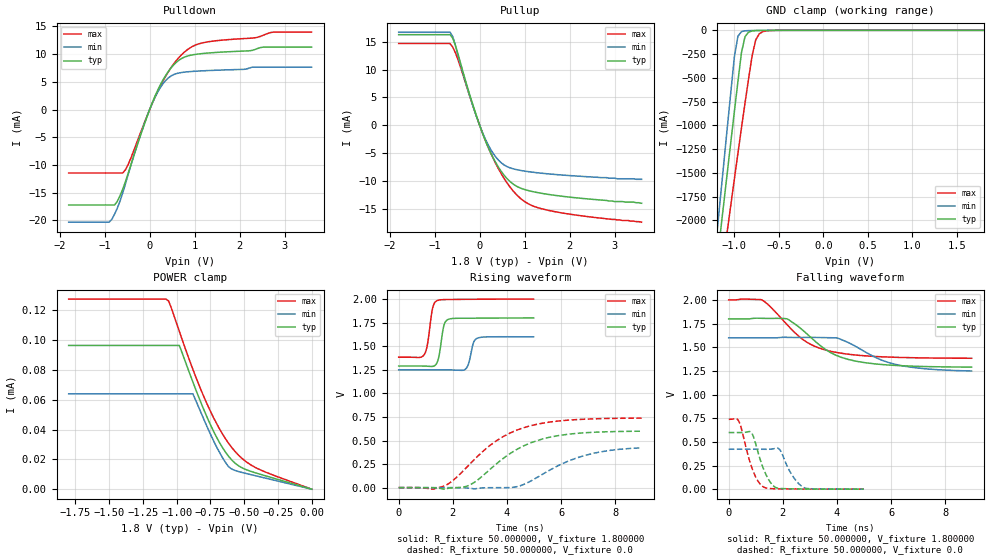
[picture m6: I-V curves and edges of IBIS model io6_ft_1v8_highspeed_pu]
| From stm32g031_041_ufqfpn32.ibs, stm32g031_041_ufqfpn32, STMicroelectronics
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|   Model io6_ft_1v8_highspeed_pu
[Model]  io6_ft_1v8_highspeed_pu
Model_type I/O
Polarity   Non-Inverting
Enable   Active-Low
Vinl =   0.540000V
Vinh =   1.260000V
Vmeas =  0.900000V
Cref =   50.000000pF
Rref =   100.000000M
Vref =   0.0V
C_comp   1.277600pF   1.236700pF   1.315100pF
[Temperature Range]   25.000000   -40.000000   0.125000k
[Pullup Reference]   1.800000V   1.600000V   2.000000V
[Pulldown Reference]   0.0V   0.0V   0.0V
[POWER Clamp Reference]   1.800000V   1.600000V   2.000000V
[GND Clamp Reference]   0.0V   0.0V   0.0V
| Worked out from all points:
|   slope of the pulldown table from 0 to 0.27 V, typ, clamps not added: 54.7 ohm
|   slope of the pullup table from 0 to 0.27 V, typ, clamps not added: 50.6 ohm
|   GND clamp passes 1 mA (typ) near -0.66 V on its own axis
|   rising waveform, R_fixture 50.000000, V_fixture 1.800000: 20-80 % time 166ps typ, 169ps min, 180ps max; typ from 1.29 V to 1.8 V
|   rising waveform, R_fixture 50.000000, V_fixture 0.0: 20-80 % time 1.83ns typ, 1.86ns min, 1.92ns max; typ from 0.001 V to 0.599 V
|   falling waveform, R_fixture 50.000000, V_fixture 1.800000: 20-80 % time 1.51ns typ, 1.6ns min, 1.49ns max; typ from 1.8 V to 1.29 V
|   falling waveform, R_fixture 50.000000, V_fixture 0.0: 20-80 % time 441ps typ, 482ps min, 451ps max; typ from 0.599 V to 0.001 V
[Pulldown]
|Voltage   I(typ)   I(min)   I(max)
-1.8V     -17.22mA   -20.33mA   -11.45mA
-900mV    -17.22mA   -20.33mA   -11.45mA
-720mV    -16.58mA   -17.82mA   -11.45mA
-600mV    -14.41mA   -15.08mA   -11.45mA
-480mV    -11.58mA   -11.79mA   -9.955mA
0V        0A         0A         0A
240mV     4.49mA     3.999mA    4.291mA
480mV     7.563mA    6.085mA    7.612mA
780mV     9.487mA    6.76mA     10.43mA
1.14V     10.08mA    6.976mA    11.96mA
2.76V     11.26mA    7.647mA    13.98mA
3.6V      11.26mA    7.647mA    13.98mA
[Pullup]
|Voltage   I(typ)   I(min)   I(max)
-1.8V     16.27mA    16.74mA    14.68mA
-660mV    16.27mA    16.74mA    14.68mA
-600mV    15.66mA    15.96mA    14.07mA
-480mV    12.75mA    12.58mA    11.77mA
-180mV    4.421mA    4.232mA    4.226mA
120mV     -2.604mA   -2.366mA   -2.563mA
420mV     -7.546mA   -6.272mA   -7.834mA
600mV     -9.499mA   -7.385mA   -10.25mA
780mV     -10.75mA   -7.883mA   -12.12mA
1.08V     -11.72mA   -8.32mA    -14.1mA
1.5V      -12.38mA   -8.703mA   -15.22mA
3.6V      -14mA      -9.7mA     -17.4mA
[GND_clamp]
|Voltage   I(typ)   I(min)   I(max)
-1.8V     -7.471A    -7.973A    -7.298A
-1.2V     -2.489A    -2.18A     -2.954A
-1.16V    -2.16A     -1.797A    -2.674A
-1.08V    -1.505A    -1.034A    -2.118A
-1V       -857.9mA   -283.1mA   -1.568A
-960mV    -540.4mA   -62.14mA   -1.296A
-920mV    -234.4mA   -13.75mA   -1.028A
-880mV    -66.29mA   -4.855mA   -765.3mA
-800mV    -6.505mA   -2.056mA   -266mA
-760mV    -3.074mA   -1.45mA    -100.4mA
-680mV    -1.215mA   -557.1uA   -14.19mA
1.8V      0A         0A         0A
[POWER_clamp]
|Voltage   I(typ)   I(min)   I(max)
-1.8V     96.34uA    63.94uA    127.5uA
-1.08V    96.34uA    63.94uA    127.5uA
-1.06V    96.34uA    63.94uA    126.3uA
-980mV    96.34uA    63.94uA    105.8uA
-880mV    71.93uA    63.94uA    80.41uA
-800mV    53.62uA    47.15uA    62.36uA
-720mV    37.64uA    31.24uA    46.77uA
-640mV    25.08uA    18.16uA    34.09uA
-600mV    20.4uA     13.93uA    28.92uA
-520mV    14.54uA    11.31uA    20.97uA
-420mV    11.06uA    9.102uA    14.71uA
0V        0A         0A         0A
[Ramp]
| variable   typ   min   max
dV/dt_r  0.34953/1.75108n   0.20693/1.41820n   0.43527/1.86936n
dV/dt_f  0.29988/1.46261n   0.18882/1.35156n   0.36630/1.46807n
R_load = 50.000000
[Rising Waveform]
R_fixture= 50.000000
V_fixture= 1.800000
V_fixture_min= 1.600000
V_fixture_max= 2.000000
|time   V(typ)   V(min)   V(max)
0s        1.29V      1.249V     1.384V
940.9ps   1.289V     1.249V     1.41V
1.061ns   1.288V     1.25V      1.516V
1.261ns   1.287V     1.25V      1.912V
1.421ns   1.329V     1.25V      1.983V
1.662ns   1.71V      1.25V      1.994V
1.822ns   1.783V     1.249V     1.995V
2.482ns   1.797V     1.261V     1.997V
2.893ns   1.797V     1.584V     1.998V
4.985ns   1.8V       1.6V       2V
[Rising Waveform]
R_fixture= 50.000000
V_fixture= 0.0
V_fixture_min= 0.0
V_fixture_max= 0.0
|time   V(typ)   V(min)   V(max)
0s        1.129mV    851.3uV    1.639mV
1.568ns   -8.999mV   844.3uV    7.949mV
1.982ns   -1.112mV   988.9uV    71.76mV
2.505ns   15.57mV    -2.566mV   214.1mV
3.622ns   255.9mV    787.1uV    499.6mV
4.324ns   399.1mV    8.83mV     605.8mV
4.757ns   461.1mV    53.01mV    648mV
6.595ns   576.5mV    317.6mV    722.5mV
7.748ns   593.5mV    393.7mV    733.9mV
8.973ns   599.2mV    422.6mV    738.1mV
[Falling Waveform]
R_fixture= 50.000000
V_fixture= 1.800000
V_fixture_min= 1.600000
V_fixture_max= 2.000000
|time   V(typ)   V(min)   V(max)
0s        1.8V       1.6V       2V
1.243ns   1.806V     1.6V       1.998V
2.162ns   1.799V     1.605V     1.738V
2.883ns   1.643V     1.604V     1.555V
3.712ns   1.453V     1.601V     1.461V
4.036ns   1.408V     1.595V     1.443V
4.739ns   1.351V     1.501V     1.417V
5.477ns   1.322V     1.385V     1.402V
6.18ns    1.308V     1.318V     1.394V
8.973ns   1.29V      1.249V     1.384V
[Falling Waveform]
R_fixture= 50.000000
V_fixture= 0.0
V_fixture_min= 0.0
V_fixture_max= 0.0
|time   V(typ)   V(min)   V(max)
0s        599.2mV    422.6mV    738.1mV
390.4ps   598.8mV    422.7mV    708.9mV
840.8ps   597.7mV    422.8mV    240.3mV
1.071ns   403.8mV    422.8mV    90.67mV
1.311ns   198mV      422.3mV    20.54mV
1.622ns   43.83mV    426.1mV    5.978mV
1.862ns   9.68mV     425.9mV    4.332mV
2.372ns   4.162mV    136.2mV    3.01mV
2.793ns   2.69mV     15.75mV    2.524mV
4.985ns   1.129mV    851.3uV    1.639mV
